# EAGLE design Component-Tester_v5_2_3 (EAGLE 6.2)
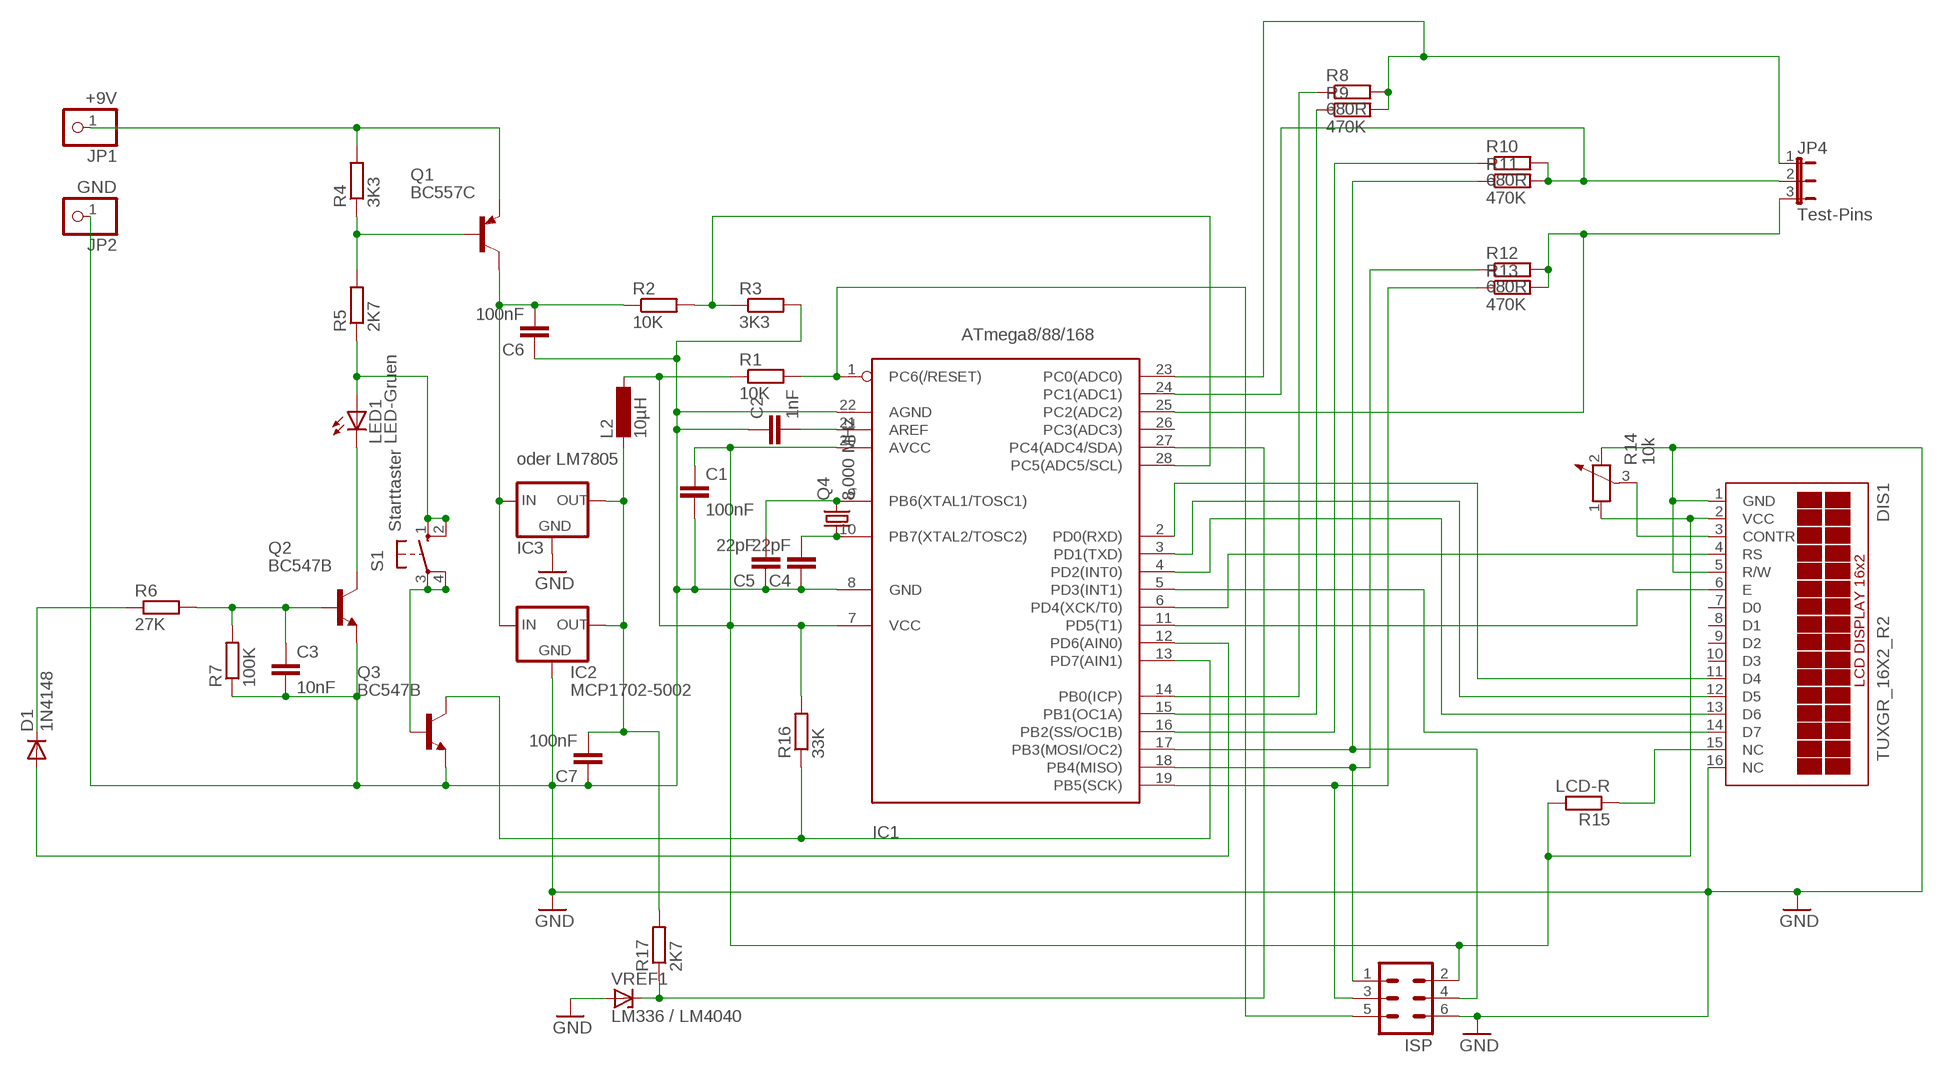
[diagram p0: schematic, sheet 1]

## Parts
C1  100nF  C-EU025_050-025X075  [C025_050-025X075]
C2  1nF  C2.5/2  [C2.5-2]
C3  10nF  C2.5/2  [C2.5-2]
C4  22pF  C2.5/2  [C2.5-2]
C5  22pF  C2.5/2  [C2.5-2]
C6  100nF  C-EU025_050-025X075  [C025_050-025X075]
C7  100nF  C-EU025_050-025X075  [C025_050-025X075]
D1  1N4148  1N4148DO35-7  [DO35-7]
DIS1  TUXGR_16X2_R2  [TUXGR_16X2_R2]
IC1  ATmega8/88/168  MEGA8-P  [DIL28-3]
IC2  MCP1702-5002  [TO92-LOWDROP]
IC3  oder LM7805  78XXL  [78XXL]
ISP  ML6L  [ML6L]
JP1  +9V  PINHD-1X1  [1X01]
JP2  GND  PINHD-1X1  [1X01]
JP4  Test-Pins  JP2E  [JP2]
L2  10µH  L-EU0207/10  [0207/10]
LED1  LED-Gruen  LED5MM  [LED5MM]
Q1  BC557C  [TO92-EBC]
Q2  BC547B  [TO92]
Q3  BC547B  [TO92]
Q4  8,000 MHz  CRYSTALHC49S  [HC49/S]
R1  10K  R-EU_0207/10  [0207/10]
R2  10K  R-EU_0207/10  [0207/10]
R3  3K3  R-EU_0207/10  [0207/10]
R4  3K3  R-EU_0207/10  [0207/10]
R5  2K7  R-EU_0207/10  [0207/10]
R6  27K  R-EU_0207/10  [0207/10]
R7  100K  R-EU_0207/10  [0207/10]
R8  680R  R-EU_0207/10  [0207/10]
R9  470K  R-EU_0207/10  [0207/10]
R10  680R  R-EU_0207/10  [0207/10]
R11  470K  R-EU_0207/10  [0207/10]
R12  680R  R-EU_0207/10  [0207/10]
R13  470K  R-EU_0207/10  [0207/10]
R14  10k  POTENTIOMETER_PT-10  [PT-10]
R15  LCD-R  R-EU_0207/10  [0207/10]
R16  33K  R-EU_0207/10  [0207/10]
R17  2K7  R-EU_0207/10  [0207/10]
S1  Starttaster  10-XX  [B3F-10XX]
VREF1  LM336 / LM4040  LM4040  [TO92-VREF]

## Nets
GND: C1.2 C2.1 C3.2 C4.1 C5.1 C6.1 C7.1 DIS1.1(GND) DIS1.5(R/W) DIS1.16(NC) IC1.8(GND) IC1.22(AGND) IC2.GND IC3.GND ISP.6 JP2.1 Q2.1(E) Q3.1(E) R3.2 R7.1 R14.2 VREF1.-
N$2: C6.2 IC2.IN IC3.IN Q1.C R2.1
N$3: IC1.1(PC6(/RESET)) ISP.5 R1.2
N$4: C2.2 IC1.21(AREF)
N$5: Q1.B R4.1 R5.2
N$6: IC1.28(PC5(ADC5/SCL)) R2.2 R3.1
N$8: C1.1 DIS1.2(VCC) IC1.7(VCC) IC1.20(AVCC) ISP.2 L2.1 R1.1 R14.1 R15.2 R16.2
N$9: LED1.K(C) Q2.3(C)
N$10: IC1.13(PD7(AIN1)) Q3.3(C) R16.1
N$11: C3.1 Q2.2(B) R6.2 R7.2
N$12: D1.A IC1.12(PD6(AIN0))
N$13: IC1.25(PC2(ADC2)) JP4.3 R12.2 R13.2
N$14: Q3.2(B) S1.3(P) S1.4(P1)
N$15: IC1.24(PC1(ADC1)) JP4.2 R10.2 R11.2
N$16: IC1.23(PC0(ADC0)) JP4.1 R8.2 R9.2
N$17: C7.2 IC2.OUT IC3.OUT L2.2 R17.2
N$18: IC1.18(PB4(MISO)) ISP.1 R12.1
N$19: IC1.14(PB0(ICP)) R8.1
N$20: IC1.15(PB1(OC1A)) R9.1
N$21: IC1.16(PB2(SS/OC1B)) R10.1
N$23: LED1.A R5.1 S1.1(S) S1.2(S1)
N$24: DIS1.3(CONTR) R14.3
N$25: DIS1.4(RS) IC1.6(PD4(XCK/T0))
N$26: DIS1.6(E) IC1.11(PD5(T1))
N$27: DIS1.11(D4) IC1.2(PD0(RXD))
N$28: DIS1.12(D5) IC1.3(PD1(TXD))
N$29: DIS1.13(D6) IC1.4(PD2(INT0))
N$30: DIS1.14(D7) IC1.5(PD3(INT1))
N$31: C4.2 IC1.10(PB7(XTAL2/TOSC2)) Q4.1
N$32: DIS1.15(NC) R15.1
N$33: JP1.1 Q1.E R4.2
N$34: C5.2 IC1.9(PB6(XTAL1/TOSC1)) Q4.2
N$37: D1.C R6.1
N$39: IC1.17(PB3(MOSI/OC2)) ISP.4 R11.1
N$40: IC1.27(PC4(ADC4/SDA)) R17.1 VREF1.+
N$42: IC1.19(PB5(SCK)) ISP.3 R13.1
Unconnected: DIS1.7(D0) DIS1.8(D1) DIS1.9(D2) DIS1.10(D3) IC1.26(PC3(ADC3))

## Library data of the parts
C1 C6 C7 = rcl:C-EU: CAPACITOR, European symbol
C2-C5 = capacitor-wima:C: CAPACITOR
D1 = diode:1N4148: DIODE
DIS1 = display-lcd:TUXGR_16X2_R2: Tuxgraphics LCD display 16x2 characters reflective, without background light Source: tuxgr_12x2_r2.pdf; OC_FARNELL: unknown; OC_NEWARK: unknown
IC1 = avr-6:MEGA8-P: MICROCONTROLLER 8 Kbytes FLASH 1 kbytes SRAM 512 bytes EEPROM USART 4-channel 10 bit ADC 2-channel 8 bit ADC
IC2 = asko:MCP1702-5002
IC3 = v-reg:78XXL: VOLTAGE REGULATOR
ISP = con-ml:ML6L: HARTING; OC_FARNELL: unknown; OC_NEWARK: unknown
JP1 JP2 = pinhead:PINHD-1X1: PIN HEADER
JP4 = jumper:JP2E: JUMPER
L2 = rcl:L-EU: INDUCTOR, European symbol
LED1 = led:LED: LED
Q1 = transistor-pnp:BC557*: PNP Transistror
Q2 Q3 = transistor-npn:BC547*: NPN Transistor
Q4 = crystal:CRYSTAL: CRYSTAL; OC_FARNELL: 1667008; OC_NEWARK: unknown
R1-R13 R15-R17 = resistor:R-EU_: RESISTOR, European symbol
R14 = rcl:POTENTIOMETER_: Potentiometer
S1 = switch-omron:10-XX: OMRON SWITCH; MPN: B3F-1000; OC_FARNELL: 176432; OC_NEWARK: 36M3542
VREF1 = asko:LM4040

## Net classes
0 default: width 0.406 mm, drill 0.8 mm

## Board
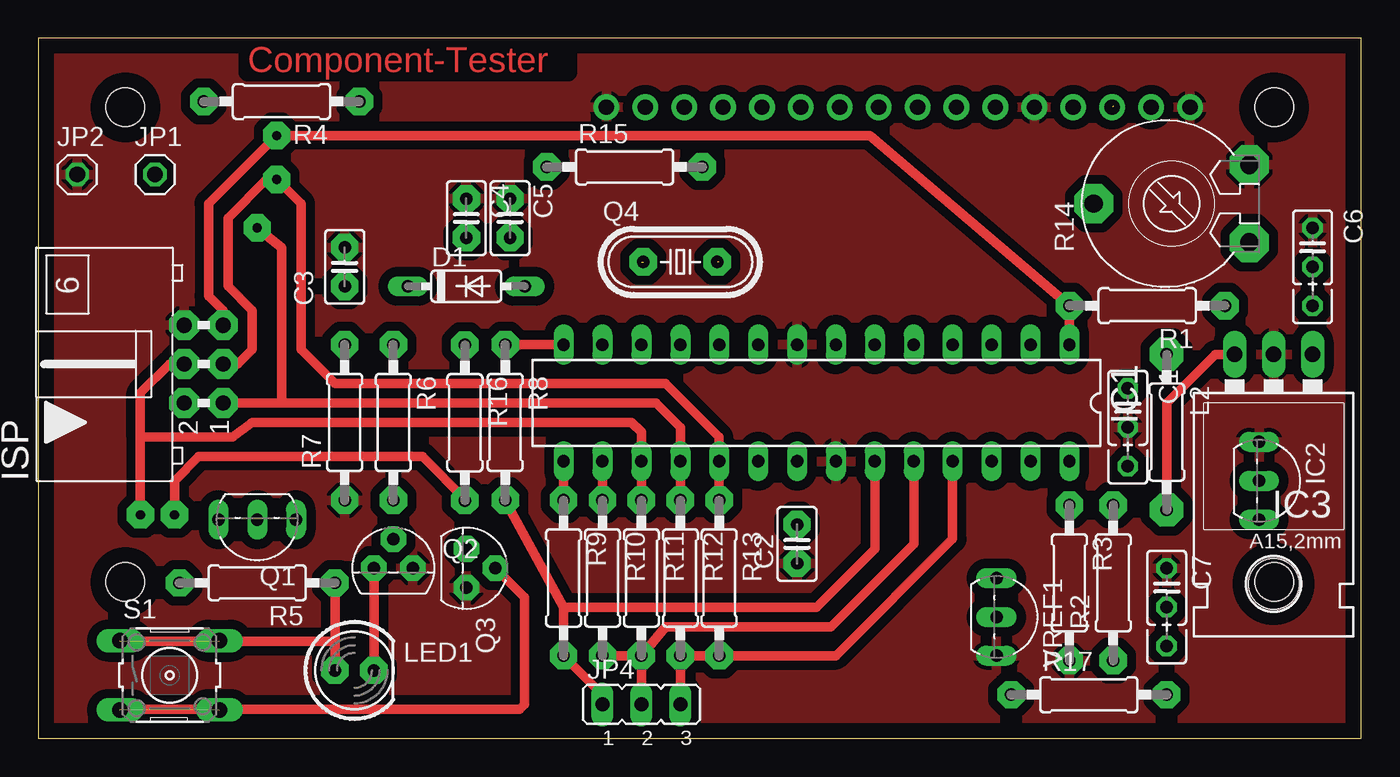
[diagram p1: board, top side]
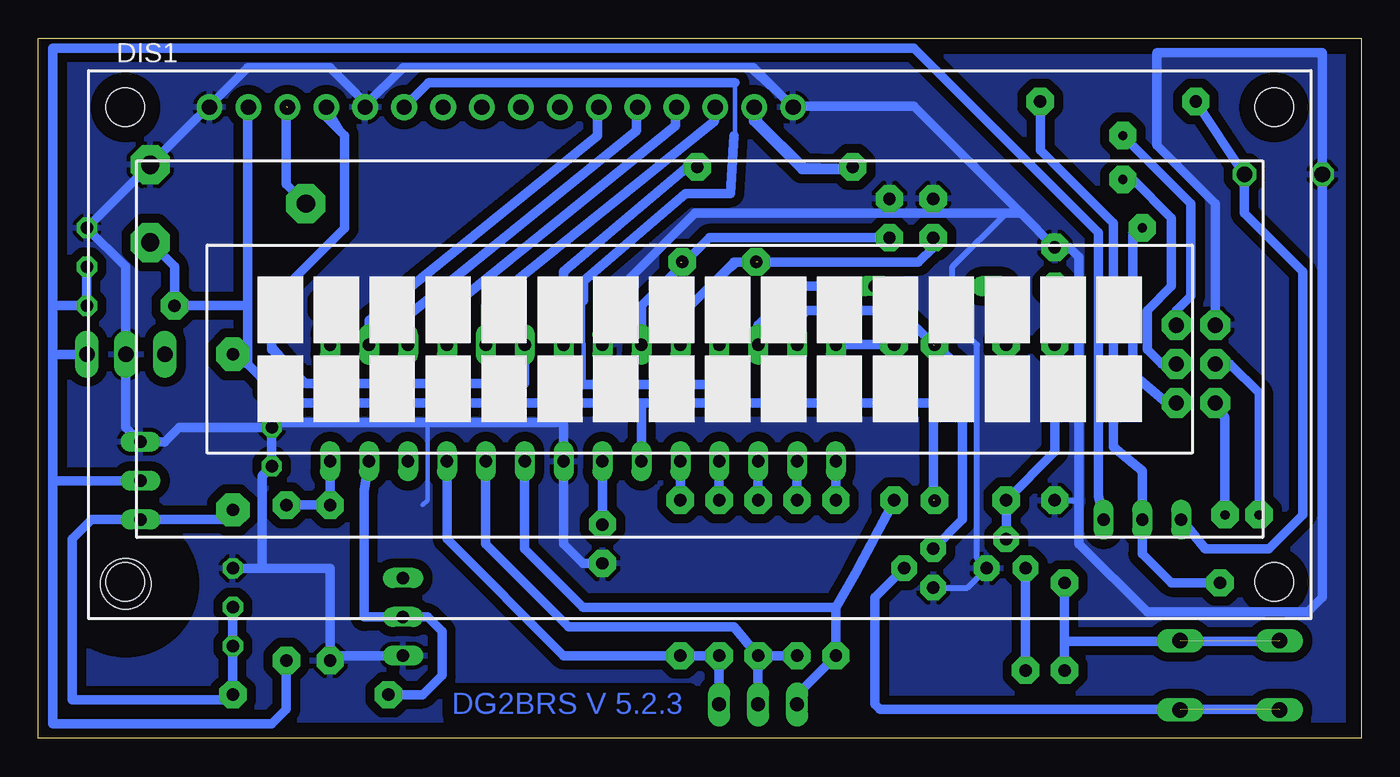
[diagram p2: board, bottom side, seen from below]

Size 86.36 x 45.72 mm. Coordinates in mm from the lower left corner, seen from the top.
Outline: 0,0 86.36,0 86.36,45.72 0,45.72 0,0
Copper layers (1*16): Top 0.035mm / dielectric 1.5mm / Bottom 0.035mm
Design rules: minimum track width 10mil, minimum drill 24mil, track to track 8mil, track to pad 8mil, pad to pad 8mil, via to via 8mil, smd to smd 8mil, copper to edge 40mil, drill to drill 8mil, minimum pad ring 10mil, minimum via ring 8mil, stop-mask expansion 4mil, vias tented up to drill 0mil, thermal gap 10mil

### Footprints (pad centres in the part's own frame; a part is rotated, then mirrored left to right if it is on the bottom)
C025_050-025X075 = drill 0.813 octagon: 1 -1.27,0; 2 1.27,0; 3 3.81,0
C2.5-2 = drill 0.813 pad 1.778 octagon: 1 -1.27,0; 2 1.27,0
DO35-7 = drill 0.813 long: A 3.81,0; C -3.81,0
TUXGR_16X2_R2 = drill 1 pad 1.676: 1 -32,15.5; 2 -29.46,15.5; 3 -26.92,15.5; 4 -24.38,15.5; 5 -21.84,15.5; 6 -19.3,15.5; 7 -16.76,15.5; 8 -14.22,15.5; 9 -11.68,15.5; 10 -9.14,15.5; 11 -6.6,15.5; 12 -4.06,15.5; 13 -1.52,15.5; 14 1.02,15.5; 15 3.56,15.5; 16 6.1,15.5 | hole 2.5: -37.5,-15.5; 37.5,-15.5; -37.5,15.5; 37.5,15.5
DIL28-3 = drill 0.813 long: 1 -16.51,-3.81; 2 -13.97,-3.81; 3 -11.43,-3.81; 4 -8.89,-3.81; 5 -6.35,-3.81; 6 -3.81,-3.81; 7 -1.27,-3.81; 8 1.27,-3.81; 9 3.81,-3.81; 10 6.35,-3.81; 11 8.89,-3.81; 12 11.43,-3.81; 13 13.97,-3.81; 14 16.51,-3.81; 15 16.51,3.81; 16 13.97,3.81; 17 11.43,3.81; 18 8.89,3.81; 19 6.35,3.81; 20 3.81,3.81; 21 1.27,3.81; 22 -1.27,3.81; 23 -3.81,3.81; 24 -6.35,3.81; 25 -8.89,3.81; 26 -11.43,3.81; 27 -13.97,3.81; 28 -16.51,3.81
TO92-LOWDROP = drill 0.813 long: GND -3.81,0; IN -1.27,0; OUT 1.27,0
78XXL = drill 1.016 long: GND 0,-3.81; IN -2.54,-3.81; OUT 2.54,-3.81 | hole 3.302: 0,11.176
ML6L = drill 1 pad 1.93 octagon: 1 -2.54,-1.27; 2 -2.54,1.27; 3 0,-1.27; 4 0,1.27; 5 2.54,-1.27; 6 2.54,1.27
1X01 = drill 1.016 octagon: 1 0,0
JP2 = drill 0.914 long: 1 -2.54,0; 2 0,0; 3 2.54,0
0207/10 = drill 0.813 pad 2.184 octagon: 1 -5.08,0; 2 5.08,0
LED5MM = drill 0.813 pad 1.778 octagon: A -1.27,0; K 1.27,0
TO92-EBC = drill 0.813 long: B 0,-1.27; C -2.54,-1.27; E 2.54,-1.27
TO92 = drill 0.813 pad 1.676 octagon: 1 1.27,0; 2 0,1.905; 3 -1.27,0
HC49/S = drill 0.813 pad 1.778 octagon: 1 -2.413,0; 2 2.413,0
0207/10' = drill 0.813 pad 1.778 octagon: 1 -5.08,0; 2 5.08,0
PT-10 = drill 1.2 pad 2.54 octagon: 1 -2.54,-5.08; 2 2.54,-5.08; 3 0,5.08
B3F-10XX = drill 1.016 long: 1 -3.251,2.261; 2 3.251,2.261; 3 -3.251,-2.261; 4 3.251,-2.261
TO92-VREF = drill 0.813 long: + 0,0; - 2.54,0; NC -2.54,0

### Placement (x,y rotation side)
C1  71.12,21.59 270 top
C2  49.53,12.7 90 top
C3  20,30.8 90 top
C4  27.94,33.97 270 top
C5  30.8,33.97 270 top
C6  83.19,32.07 270 top
C7  73.66,9.84 270 top
D1  27.94,29.53 0 top
DIS1  43.18,25.72 0 bottom
IC1  50.8,21.91 180 top
IC2  79.69,15.56 270 top
IC3  80.64,21.27 180 top
ISP  10.79,24.45 90 top
JP1  7.62,36.83 0 top
JP2  2.54,36.83 0 top
JP4  39.37,2.22 0 top
L2  73.66,20 270 top
LED1  20.64,4.45 0 top
Q1  14.29,13.02 180 top
Q2  23.18,11.11 0 top
Q3  27.94,11.11 270 top
Q4  41.91,31.11 0 top
R1  10K  [0207/10']  72.39,28.26 180 top
R2  10K  [0207/10']  70.17,10.16 90 top
R3  3K3  [0207/10']  67.31,10.16 270 top
R4  3K3  [0207/10']  15.88,41.59 180 top
R5  2K7  [0207/10']  14.29,10.16 180 top
R6  27K  [0207/10']  23.18,20.64 270 top
R7  100K  [0207/10']  20,20.64 90 top
R8  680R  [0207/10']  30.48,20.64 270 top
R9  470K  [0207/10']  34.29,10.48 270 top
R10  680R  [0207/10']  36.83,10.48 270 top
R11  470K  [0207/10']  39.37,10.48 270 top
R12  680R  [0207/10']  41.91,10.48 270 top
R13  470K  [0207/10']  44.45,10.48 270 top
R14  73.98,34.93 90 top
R15  LCD-R  [0207/10']  38.27,37.32 0 top
R16  33K  [0207/10']  27.84,20.61 270 top
R17  2K7  [0207/10']  68.58,2.86 0 top
S1  8.57,4.13 0 top
VREF1  62.55,7.94 270 top

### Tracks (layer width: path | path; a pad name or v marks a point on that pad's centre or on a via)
GND
  Bottom 0.305: 60.96,20.64 60.96,15.56 61.28,15.24
  Bottom 0.406: 62.23,43.82 40.01,43.82 36.83,40.96 DIS1.16 | 20.32,15.56 R7.1 18.41,15.56 | Q3.1 25.72,9.84 Q2.1 25.08,11.75 25.08,25.72 26.67,27.31 26.67,30.8 23.18,34.29
  Bottom 0.61: 22.22,34.29 23.18,34.29 43.5,34.29 49.53,28.26 IC1.8 | 22.22,34.29 29.21,41.28 37.15,41.28 39.69,43.82 62.55,43.82 65.09,41.28 65.09,41.59 67.31,43.82 72.71,43.82 R14.2 C6.1 80.64,30.8 IC3.GND 80.64,20.32 IC2.GND 78.1,19.37 77.15,20.32 C1.2 | 22.22,34.29 C3.2 19.05,32.07 18.41,31.43 18.41,15.56 18.41,12.7 13.97,8.26 3.49,8.26 2.54,9.21 JP2.1 2.54,44.77 13.33,44.77 13.33,38.73 9.53,34.93 ISP.6 | VREF1.- 66.99,5.4 | 67.31,5.4 R3.2 67.31,11.11 71.75,11.11 | 71.75,11.11 71.75,17.15 71.12,17.78 C1.2 | C2.1 50.8,11.43 52.07,12.7 IC1.22 52.07,20.64 60.96,20.64 70.8,20.64 C1.2 | C7.1 71.75,11.11
  pour Bottom (isolate 0.61): -0.32,46.67 86.68,46.36 86.68,-0.64 -0.32,-0.32
  pour Top (isolate 0.61): 0,46.67 86.68,46.36 86.68,-0.64 -0.32,-0.32
N$1  (via drill 0.8)
  other vias: 5.71,41.28
N$2
  Bottom 0.406: Q1.C 17.14,15.56 17.14,15.87
  Bottom 0.61: 85.41,28.26 85.41,45.08 29.21,45.08 17.14,33.02 17.14,15.87 Q1.C | 85.41,16.83 85.41,0.95 71.12,0.95 70.17,1.9 R2.1 | 85.41,28.26 83.19,28.26 C6.2 | 85.41,28.26 85.41,25.08 | 85.41,25.08 85.41,16.83 | 85.41,16.83 IC2.IN | IC3.IN 85.41,25.08
N$3  (via drill 0.6 pad 1.78)
  Top 0.61: ISP.5 12.06,27.94 11.11,28.89 11.11,34.93 v15.56,39.37 54.29,39.37 R1.2 IC1.1
  Bottom 0.61: IC1.1 R1.2 | v15.56,39.37 11.11,34.93 11.11,28.89 12.06,27.94 ISP.5
N$4
  Bottom 0.61: IC1.21 C2.2
N$5
  Bottom 0.61: R4.1 20.95,38.42 16.19,33.65 16.19,19.05 14.29,17.46 Q1.B 14.29,12.07 12.38,10.16 R5.2
N$6
  Bottom 0.61: IC1.28 R3.1 R2.2
N$7  (via drill 0.8)
  other vias: 5.71,10.16
N$8  (via drill 0.6 pad 1.78)  (2 unrouted)
  Top 0.61: 27.94,15.56 25.08,18.42 10.48,18.42 8.89,16.83 v8.89,14.6
  Bottom 0.406: 72.71,28.26 72.71,40.96 DIS1.2 | 43.89,37.39 R15.2 | R14.1 79.06,32.07
  Bottom 0.61: 43.89,37.39 52.07,30.48 IC1.7 52.07,21.91 | 46.99,21.91 IC1.20 | 27.94,15.56 27.94,21.91 46.99,21.91 | 46.99,21.91 52.07,21.91 | 72.71,24.45 L2.1 | 72.71,24.45 C1.1 70.17,21.91 52.07,21.91 | 72.71,24.45 72.71,28.26 | 72.71,28.26 72.71,41.28 | R14.1 77.47,30.8 R1.1 72.71,28.26 | ISP.2 8.89,20.95 v8.89,14.6
N$9
  Top 0.61: Q2.3 LED1.K
  Bottom 0.61: Q2.3 LED1.K
N$10  (1 unrouted)
  Bottom 0.61: Q3.3 26.04,14.29 26.04,24.13 27.94,25.72 30.16,27.94 36.2,27.94 36.83,27.31 IC1.13
N$11
  Bottom 0.406: C3.1 R7.2 20,18.73
  Bottom 0.61: Q2.2 R6.2 20,18.73 C3.1
N$12
  Bottom 0.61: D1.A 36.83,29.53 39.37,26.99 IC1.12
N$13
  Top 0.406: IC1.25 59.69,14.29
  Top 0.61: JP4.3 R12.2 R13.2 52.07,5.4 59.69,13.02 IC1.25
  Bottom 0.61: JP4.3 R12.2 R13.2 52.07,5.4 59.69,13.02 IC1.25
N$14  (2 unrouted)
  Top 0.61: Q3.2 31.75,9.21 31.75,2.22 31.43,1.9 5.4,1.9
  Bottom 0.61: Q3.2 31.75,9.21 31.75,2.22 31.43,1.9 5.4,1.9
N$15
  Top 0.406: IC1.24 57.15,13.65
  Top 0.61: R10.2 R11.2 | R11.2 JP4.2 | R11.2 40.96,7.3 51.75,7.3 57.15,12.7 IC1.24
  Bottom 0.61: R10.2 R11.2 | R11.2 JP4.2 | R11.2 40.96,7.3 51.75,7.3 57.15,12.7 IC1.24
N$16
  Top 0.406: 36.83,2.86 JP4.1
  Top 0.61: 36.83,2.86 R9.2 34.29,8.57 | R8.2 34.29,8.57 | 34.29,8.57 50.8,8.57 54.61,12.38 IC1.23
  Bottom 0.406: 34.29,8.57 R8.2
  Bottom 0.61: 34.29,8.57 50.8,8.57 54.61,12.38 IC1.23 | JP4.1 36.83,2.86 R9.2 34.29,8.57 | 34.29,8.57 33.02,10.79 R8.2
N$17
  Top 0.61: IC3.OUT 76.83,25.08 73.66,21.91 L2.2
  Bottom 0.61: L2.2 74.3,14.29 IC2.OUT 82.87,14.29 84.14,13.02 84.14,2.54 73.98,2.54 R17.2 C7.2
N$18  (via drill 0.6 pad 1.78)
  Top 0.61: R12.1 IC1.18 41.91,20.32 40.32,21.91 15.88,21.91 | ISP.1 15.88,21.91 | v14.29,33.34 15.88,32.07 15.88,21.91
  Bottom 0.61: IC1.18 R12.1 | ISP.1 12.7,21.91 14.92,23.81 14.92,33.02 v14.29,33.34
N$19
  Top 0.61: IC1.14 R8.1
  Bottom 0.61: IC1.14 R8.1
N$20
  Top 0.61: IC1.15 R9.1
  Bottom 0.61: IC1.15 R9.1
N$21
  Top 0.61: IC1.16 R10.1
  Bottom 0.61: IC1.16 R10.1
N$23  (2 unrouted)
  Top 0.61: 5.4,6.35 19.37,6.35 | 19.37,6.35 LED1.A | 19.37,6.35 R5.1
  Bottom 0.61: LED1.A 19.37,6.35 | 19.37,6.35 R5.1 | 5.4,6.35 19.37,6.35
N$24  (1 unrouted)
  Bottom 0.61: R14.3 70.17,36.19 70.17,41.28
N$25
  Bottom 0.406: 68.9,23.18 71.12,25.72 71.12,28.58 71.12,28.89 | 66.36,39.37 67.31,40.96 DIS1.4
  Bottom 0.61: 67.63,41.28 67.63,40.64 66.36,39.37 66.36,33.34 71.12,28.58 71.12,25.4 68.9,23.18 54.61,23.18 IC1.6
N$26
  Bottom 0.305: 50.77,23.12 50.8,28.58 | 40.87,39.46 40.87,42.82
  Bottom 0.406: 41.91,24.18 IC1.11 | 50.8,28.58 50.77,28.61 | 40.96,39.37 40.87,39.46
  Bottom 0.61: 41.91,24.18 42.02,23.12 50.77,23.12 | 50.77,28.61 50.77,29.88 44.11,35.59 41.19,35.59 40.96,39.37 | 40.87,42.82 60.88,42.82 DIS1.6 | IC1.11 41.91,23.18
N$27
  Bottom 0.406: DIS1.11 49.85,39.37
  Bottom 0.61: 49.85,41.28 49.85,39.37 64.77,27.31 IC1.2
N$28
  Bottom 0.406: DIS1.12 47.31,39.69
  Bottom 0.61: IC1.3 62.23,27.62 47.31,39.69 47.31,41.28
N$29
  Bottom 0.406: DIS1.13 44.77,40.01
  Bottom 0.61: IC1.4 59.69,27.94 44.77,40.01 44.77,41.28
N$30
  Bottom 0.406: DIS1.14 42.23,40.32
  Bottom 0.61: IC1.5 57.15,28.26 42.23,40.32 42.23,41.28
N$31  (1 unrouted)
  Bottom 0.406: 44.45,27.62 40.96,30.8 40.64,31.11
  Bottom 0.61: C4.2 27.94,32.07 28.89,31.11 39.37,31.11 40.64,31.11 40.96,31.11 44.45,27.62 IC1.10
N$32
  Bottom 0.406: R15.1 36.35,37.39 39.27,40.32 39.27,40.87 DIS1.15
N$33
  Bottom 0.61: R4.2 JP1.1 7.62,34.29 3.81,30.48 3.81,14.6 6.03,12.38 10.16,12.38 Q1.E
N$34  (1 unrouted)
  Bottom 0.61: C5.2 42.55,32.7 44.13,31.11 | 44.13,31.11 46.99,28.26 IC1.9 | 44.45,31.11 44.13,31.11
N$35  (via drill 0.8)
  other vias: 80.64,10.16
N$36  (via drill 0.8)
  other vias: 80.64,41.28
N$37
  Bottom 0.406: D1.C 23.18,28.89 R6.1
  Bottom 0.61: R6.1 23.18,28.58 D1.C
N$38
  Bottom 0.61: 33.02,37.15 36.51,37.15 39.69,40.32 39.69,41.28
N$39  (via drill 0.6 pad 1.78)
  Top 0.61: R11.1 IC1.17 39.37,20 38.74,20.64 13.97,20.64 12.7,19.68 6.67,19.68 | 6.67,19.68 6.67,22.54 8.57,24.45 ISP.4 | 6.67,19.68 v6.67,14.6
  Bottom 0.61: IC1.17 R11.1 | ISP.4 8.57,24.45 6.67,22.54 v6.67,14.6
N$40
  Bottom 0.61: IC1.27 65.09,16.19 65.09,7.94 VREF1.+ 60.96,7.94 60.01,6.99 60.01,4.13 61.28,2.86 R17.1
N$42  (via drill 0.6 pad 1.78)
  Top 0.61: R13.1 IC1.19 44.45,19.68 40.96,23.18 19.37,23.18 17.14,25.4 17.14,34.93 v15.56,36.51 14.92,36.51 12.38,33.97 12.38,29.53 13.97,27.94 13.97,25.4 13.02,24.45 ISP.3
  Bottom 0.61: IC1.19 R13.1 | ISP.3 13.02,24.45 13.97,25.4 13.97,27.94 12.38,29.53 12.38,33.97 14.92,36.51 v15.56,36.51

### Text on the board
Top: Component-Tester
Bottom: DG2BRS V 5.2.3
